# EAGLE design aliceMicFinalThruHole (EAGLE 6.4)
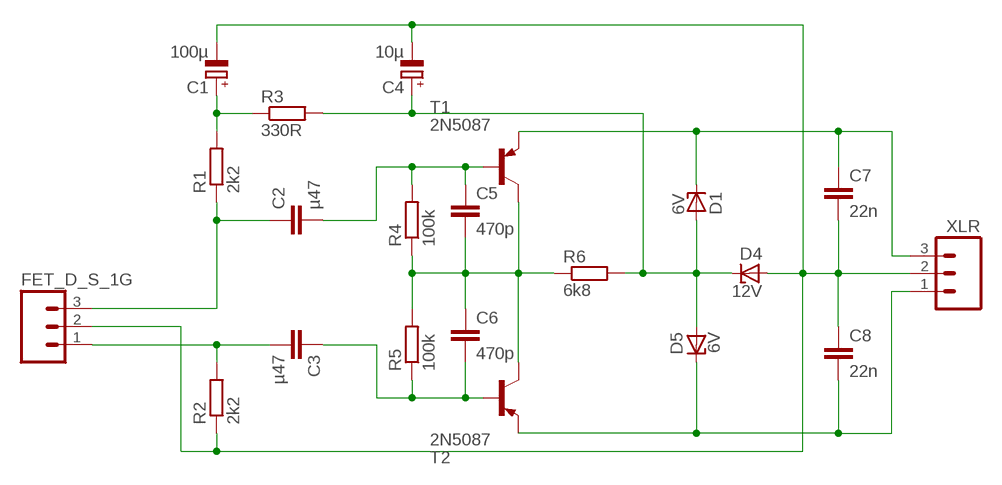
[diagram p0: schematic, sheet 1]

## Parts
C1  100µ  CPOL-EUE3.5-8  [E3,5-8]
C2  µ47  C-EU050-045X075  [C050-045X075]
C3  µ47  C-EU050-045X075  [C050-045X075]
C4  10µ  CPOL-EUE2-4  [E2-4]
C5  470p  C-EU025-024X044  [C025-024X044]
C6  470p  C-EU025-024X044  [C025-024X044]
C7  22n  C-EU025-024X044  [C025-024X044]
C8  22n  C-EU025-024X044  [C025-024X044]
D1  6V  ZENER-DIODEZD-5-SMALLSILK  [ZD-5-SMALLSILK]
D4  12V  ZENER-DIODEZD-5-SMALLSILK  [ZD-5-SMALLSILK]
D5  6V  ZENER-DIODEZD-5-SMALLSILK  [ZD-5-SMALLSILK]
FET_D_S_1G  M033.5MM-PADS  [3.5MM_PADS]
R1  2k2  R-EU_0207/2V  [0207/2V]
R2  2k2  R-EU_0207/2V  [0207/2V]
R3  330R  R-EU_0207/2V  [0207/2V]
R4  100k  R-EU_0207/2V  [0207/2V]
R5  100k  R-EU_0207/2V  [0207/2V]
R6  6k8  R-EU_0207/2V  [0207/2V]
T1  2N5087  2N5087-PNP-TO92-EBC  [TO92-EBC]
T2  2N5087  2N5087-PNP-TO92-EBC  [TO92-EBC]
XLR  M033.5MM-PADS  [3.5MM_PADS]

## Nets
GND: C1.- C4.- C7.2 C8.1 D4.A FET_D_S_1G.2 R2.1 XLR.2
N$2: C4.+ D1.A D4.C D5.A R3.2 R6.2
N$3: C5.2 C6.1 R4.1 R5.2 R6.1 T1.C T2.C
N$4: C7.1 D1.C T1.E XLR.3
N$5: C8.2 D5.C T2.E XLR.1
N$6: C2.2 C5.1 R4.2 T1.B
N$7: C3.1 C6.2 R5.1 T2.B
N$10: C1.+ R1.2 R3.1
N$11: C2.1 FET_D_S_1G.3 R1.1
N$12: C3.2 FET_D_S_1G.1 R2.2

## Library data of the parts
C1 C4 = resistor:CPOL-EU: POLARIZED CAPACITOR, European symbol
C2 C3 = shum:C-EU: CAPACITOR, European symbol
C5-C8 = resistor:C-EU: CAPACITOR, European symbol
D1 D4 D5 = shum:ZENER-DIODE: Z-Diode
FET_D_S_1G XLR = shum:M03: Header 3 Standard 3-pin 0.1" header. Use with straight break away headers (SKU : PRT-00116), right angle break away headers (PRT-00553), swiss pins (PRT-00743), machine pins (PRT-00117), and female headers (PRT-00115). Molex polarized connector foot print use with SKU : PRT-08232 with associated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
R1-R6 = resistor:R-EU_: RESISTOR, European symbol
T1 T2 = transistor-neu-to92:*-PNP-: PNP Transistror

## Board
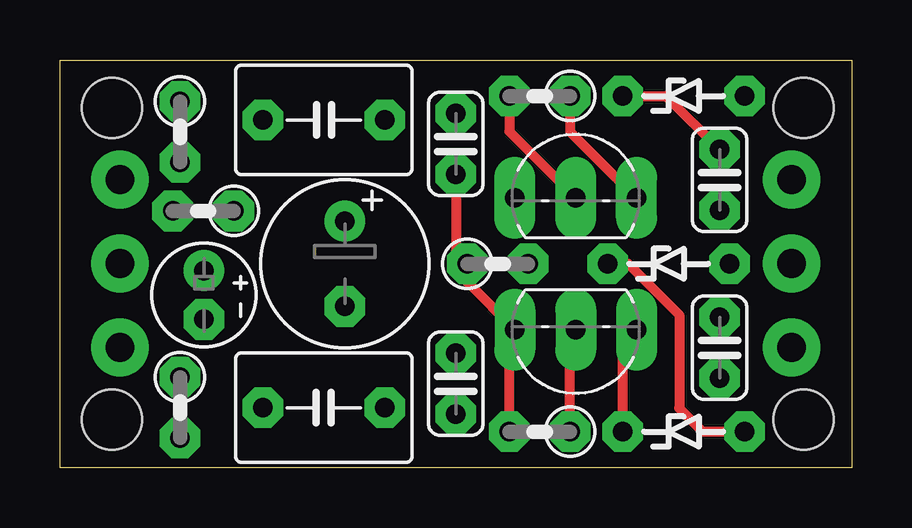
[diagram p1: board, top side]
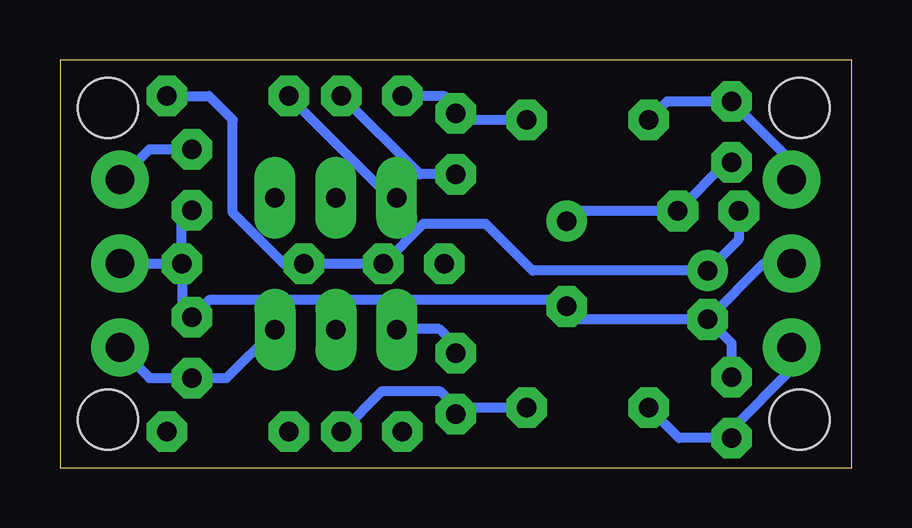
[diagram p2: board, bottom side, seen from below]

Size 33 x 17 mm. Coordinates in mm from the lower left corner, seen from the top.
Outline: 0,17 33,17 33,0 0,0 0,17
Copper layers (1*16): Top 0.035mm / dielectric 1.5mm / Bottom 0.035mm
Design rules "hackvana *": minimum track width 8mil, minimum drill 0.3mm, track to track 6mil, track to pad 6mil, pad to pad 6mil, via to via 6mil, smd to smd 0mil, copper to edge 6mil, drill to drill 6mil, minimum pad ring 17.5mil, minimum via ring 6mil, stop-mask expansion 2mil, vias tented up to drill 100mil, thermal gap 10mil
Holes 2.5 mm at 2.16,2 2.16,15 31,15 31,2

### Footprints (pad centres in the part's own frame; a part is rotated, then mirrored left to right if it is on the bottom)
E3,5-8 = drill 0.813 pad 1.6: + -1.778,0 | drill 0.813 pad 1.6 octagon: - 1.778,0
C050-045X075 = drill 0.813 octagon: 1 -2.54,0; 2 2.54,0
E2-4 = drill 0.813 pad 1.27: + -1.016,0 | drill 0.813 pad 1.27 octagon: - 1.016,0
C025-024X044 = drill 0.813 octagon: 1 -1.27,0; 2 1.27,0
ZD-5-SMALLSILK = drill 0.813 octagon: A 2.54,0; C -2.54,0
3.5MM_PADS = drill 1.2 pad 2.413: 1 -3.493,0; 2 0.007,0; 3 3.507,0
0207/2V = drill 0.813 octagon: 1 -1.27,0; 2 1.27,0
TO92-EBC = drill 0.813 long: B 0,0; C 2.54,0; E -2.54,0

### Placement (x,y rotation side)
C1  11.88,8.5 270 top
C2  11,14.5 0 top
C3  11,2.5 180 top
C4  6,7.2 270 top
C5  16.5,13.5 270 top
C6  16.5,3.5 270 top
C7  27.5,12 270 top
C8  27.5,5 270 top
D1  26,15.5 0 top
D4  25.38,8.5 0 top
D5  26,1.5 0 top
FET_D_S_1G  2.5,8.5 90 top
R1  5,14 270 top
R2  5,2.5 270 top
R3  5.97,10.7 180 top
R4  20,15.5 180 top
R5  20,1.5 180 top
R6  18.25,8.5 0 top
T1  21.5,11.25 0 top
T2  21.5,5.75 180 top
XLR  30.5,8.5 90 top

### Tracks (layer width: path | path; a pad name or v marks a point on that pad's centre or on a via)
GND
  Bottom 0.406: XLR.2 27.92,8.51 | 27.92,8.51 D4.A 27.91,6.68 C8.1 26.79,6.99 12.06,6.99 11.88,6.79 C1.- 11.34,6.18 C4.- | 27.92,8.51 27.92,10.31 C7.2 | FET_D_S_1G.2 3.68,8.51 C4.- | R2.1 5,5.18 C4.-
N$2
  Top 0.406: D4.C 23.69,8.5 25.82,6.37 25.82,2.48 26.78,1.52 28.52,1.52 D5.A
  Bottom 0.406: R3.2 4.71,9.51 C4.+ 13.3,8.22 15.24,10.16 17.86,10.16 R6.2 D4.C 23.66,8.5 25.8,10.64 25.8,14.51 26.79,15.5 D1.A
N$3
  Top 0.406: C5.2 16.5,8.98 R6.1 16.98,7.73 T2.C 18.73,5.52 R5.2 | R4.1 21.27,14.02 T1.C
  Bottom 0.406: C5.2 18,12.23 R4.1 | C6.1 16.5,5.1 17.18,5.78 18.93,5.78 T2.C
N$4
  Top 0.406: D1.C 25.27,15.5 C7.1
  Bottom 0.406: T1.E 19.21,11.25 D1.C | XLR.3 30.5,12.04 29.26,13.27 C7.1
N$5
  Top 0.406: D5.C 23.46,5.17 T2.E
  Bottom 0.406: XLR.1 30.5,4.97 29.26,3.74 C8.2 26.06,3.73 T2.E
N$6
  Top 0.406: R4.2 18.73,14.02 T1.B
  Bottom 0.406: C2.2 16.23,14.5 C5.1 16.5,15.04 16.94,15.48 18.71,15.48 R4.2
N$7
  Top 0.406: R5.1 21.27,5.52 T2.B
  Bottom 0.406: C3.1 16.23,2.5 C6.2 16.5,2.53 17.14,3.17 19.59,3.17 R5.1
N$10
  Bottom 0.406: C1.+ 11.45,10.7 R3.1 5.21,12.73 R1.2
N$11
  Bottom 0.406: FET_D_S_1G.3 2.5,12.77 R1.1 7.69,15.27 C2.1
N$12
  Bottom 0.406: C3.2 7.19,1.23 R2.2 5,1.59 2.5,4.09 FET_D_S_1G.1

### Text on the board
tValues: XLR3 | FET.S | XLR1 | 1GΩ | XLR2 | FET.D
bValues: AliceMic v.0.1 | alexanderhosford@gmail.com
